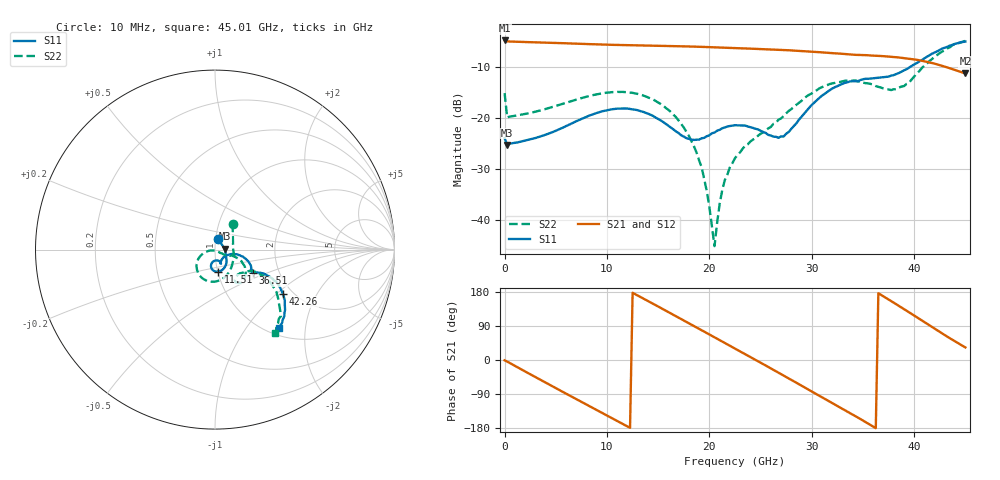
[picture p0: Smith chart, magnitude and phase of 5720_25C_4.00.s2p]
! Device:  ADRF5720
! Description: 0.5dB LSB GaAs MMIC 6-bit Digital Attenuator
! Frequency:  0.000009 -  40 GHz
! Ports:
!	RF1	= Port 1
!	RF2	= Port 2
! Vdd:  3.3 Volt
! Vss:  -3.3 Volt
! Control:  0/3.3 Volt
! State:  4.00 dB attenuation
! Data:  The device was measured using G-S-G Probes on a matrix board.
!  Data was collected using an calibrated 4 port network analyzer.
!  The reference plane for this measurement is at the launchers.
! Note:  Analog Devices supplies this data as a sample of measured data
!  for this product.  Your particular data for this product may vary.
!  Data was taken at 25 degrees C.
!  Analog Devices reserves the right to change this data at anytime.
# GHZ S DB R 45.0
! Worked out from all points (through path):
!   181 points, 10 MHz to 45.01 GHz, reference 45 ohm
!   highest |S21| = -4.77 dB at 10 MHz (marker M1); lowest = -11.3 dB at 45.01 GHz (marker M2)
!   group delay of S21, straight-line fit = 42 ps
!   lowest |S11| = -25.3 dB at 260 MHz (marker M3), VSWR 1.11, Z = 50.1 + j0.434 ohm
!   |S11| at or under -10 dB: start of sweep to 39.6 GHz
!   |S22| runs from -45.2 to -4.9 dB; largest |S21 - S12| = 0.00069
!   S11 on the Smith chart (normalised r, x): 10 MHz: 1.02, +0.13; 11.51 GHz: 1.01, -0.25; 36.51 GHz: 1.46, -0.41; 42.26 GHz: 1.78, -1.10; 45.01 GHz: 1.12, -1.44
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0.01  -24.00 75.4  -4.77 -0.9  -4.78 -0.9  -15.13 56.0
0.26  -25.31 4.6  -4.96 -4.1  -4.96 -4.1  -19.91 0.9
2.26  -24.36 -15.6  -5.09 -33.9  -5.09 -33.9  -19.13 -19.8
4.26  -23.13 -29.2  -5.22 -63.2  -5.22 -63.2  -18.11 -37.8
7.76  -19.98 -51.2  -5.45 -114.1  -5.45 -114.1  -15.96 -67.2
11.51  -18.15 -81.2  -5.68 -168.2  -5.68 -168.2  -14.89 -101.6
15.26  -20.50 -103.7  -5.83 137.4  -5.83 137.4  -17.28 -138.7
17.26  -23.43 -98.8  -5.92 108.0  -5.92 108.0  -21.20 -157.2
18.76  -24.29 -82.0  -6.00 85.8  -6.00 85.9  -26.84 -166.7
19.76  -23.61 -71.7  -6.07 71.0  -6.07 71.0  -34.47 -164.8
20.51  -22.89 -67.9  -6.12 59.9  -6.12 59.9  -45.24 -86.1
21.26  -22.05 -66.2  -6.17 48.8  -6.17 48.8  -34.25 -37.5
22.76  -21.46 -67.4  -6.29 26.5  -6.29 26.5  -27.29 -28.8
25.01  -22.54 -64.7  -6.46 -7.1  -6.46 -7.0  -23.12 -27.2
27.26  -23.66 -34.4  -6.65 -41.1  -6.65 -41.0  -19.65 -18.7
30.26  -16.97 -12.8  -7.01 -87.0  -7.01 -86.9  -14.81 -27.9
33.51  -12.99 -26.3  -7.48 -136.7  -7.48 -136.7  -12.66 -47.9
36.51  -12.12 -31.9  -7.80 176.2  -7.81 176.2  -13.90 -56.8
37.76  -11.70 -29.7  -7.98 155.7  -7.98 155.7  -14.53 -47.6
40.26  -9.22 -26.6  -8.57 113.0  -8.57 113.0  -11.31 -27.6
42.26  -6.90 -33.2  -9.48 78.1  -9.48 78.2  -7.62 -34.6
45.01  -4.98 -51.0  -11.26 33.1  -11.26 33.2  -4.86 -54.1
